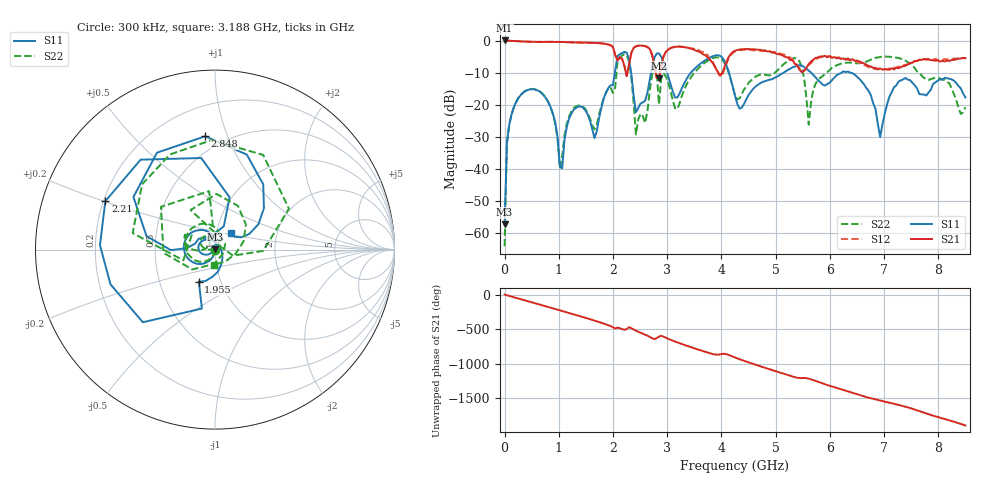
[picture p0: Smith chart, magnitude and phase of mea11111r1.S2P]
!Agilent Technologies,E5071B,MY42402595,A.08.01
!Date: Mon Jan 01 02:16:23 2001
!Data & Calibration Information:
!Freq	S11:SOLT2(ON)	S21:SOLT2(ON)	S12:SOLT2(ON)	S22:SOLT2(ON)
# Hz S dB R 50
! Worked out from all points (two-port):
!   201 points, 300 kHz to 8.5 GHz, reference 50 ohm
!   highest |S21| = 0.04 dB at 300 kHz (marker M1); lowest = -11.7 dB at 2.848 GHz (marker M2)
!   |S21| within 3 dB of the highest: start of sweep to 2.015 GHz; 3.006 GHz to 3.509 GHz (503.3 MHz wide, 15.5 % of centre)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
!   lowest |S11| = -57.2 dB at 300 kHz (marker M3), VSWR 1.00, Z = 50.1 + j0.0983 ohm
!   |S11| at or under -10 dB: start of sweep to 2.035 GHz; 4.138 GHz to 5.145 GHz (1.007 GHz wide, 21.7 % of centre); 6.383 GHz to end of sweep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
!   |S22| runs from -64.0 to -4.3 dB; largest |S21 - S12| = 0.063
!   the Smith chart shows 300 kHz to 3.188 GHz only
!   S11 on the Smith chart (normalised r, x): 300 kHz: 1.00, +0.00; 1.955 GHz: 0.78, -0.29; 2.21 GHz: 0.21, +0.20; 2.848 GHz: 0.40, +0.84; 3.188 GHz: 1.18, +0.22
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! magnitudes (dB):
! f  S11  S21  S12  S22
! 300 kHz  -57.2  0.0  0.0  -64.0
! 42.8 MHz  -32.0  0.0  0.0  -31.9
! 255.3 MHz  -17.8  -0.2  -0.2  -17.8
! 765.3 MHz  -18.0  -0.4  -0.4  -17.9
! 1.02 GHz  -39.2  -0.4  -0.4  -39.9
! 1.445 GHz  -20.9  -0.6  -0.6  -20.6
! 1.658 GHz  -30.3  -0.7  -0.7  -27.7
! 1.955 GHz  -13.9  -1.4  -1.5  -14.5
! 2.21 GHz  -3.5  -7.8  -8.0  -4.3
! 2.423 GHz  -22.3  -1.8  -1.8  -29.3
! 2.763 GHz  -5.3  -7.7  -7.5  -8.3
! 2.848 GHz  -4.0  -11.7  -11.7  -19.8
! 3.188 GHz  -17.7  -1.9  -1.9  -21.3
! 3.868 GHz  -4.7  -7.6  -7.9  -5.3
! 4.25 GHz  -17.2  -3.2  -3.4  -17.0
! 5.398 GHz  -7.7  -7.8  -7.7  -5.6
! 5.61 GHz  -9.3  -7.4  -7.5  -26.2
! 5.695 GHz  -10.7  -5.9  -6.1  -15.2
! 6.46 GHz  -10.6  -6.3  -6.3  -7.0
! 6.928 GHz  -30.0  -8.7  -8.9  -5.1
! 7.098 GHz  -17.5  -9.1  -8.7  -5.0
! 8.5 GHz  -17.7  -5.4  -5.6  -20.8
